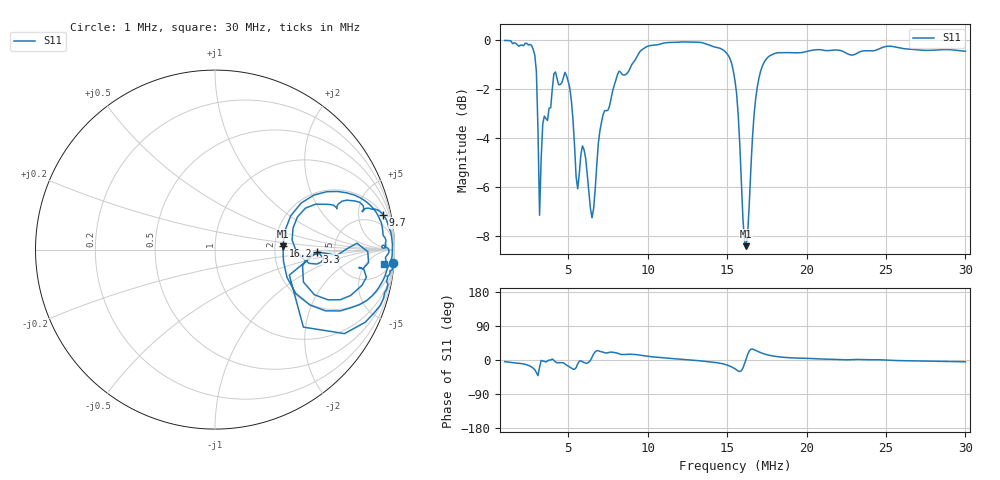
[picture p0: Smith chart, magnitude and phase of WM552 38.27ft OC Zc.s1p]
!Created via Zplots "Save as S1P" button
!Original data file:  $remote$.s1p
!Transmission line transform:  None
# MHZ S MA R 50
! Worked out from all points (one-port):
!   291 points, 1 MHz to 30 MHz, reference 50 ohm
!   lowest |S11| = -8.4 dB at 16.2 MHz (marker M1), VSWR 2.22, Z = 111 + j4.8 ohm
!   |S11| at or under -10 dB: nowhere
!   S11 on the Smith chart (normalised r, x): 1 MHz: 2, -27; 3.3 MHz: 3.65, -0.14; 9.7 MHz: 2.10, +9.36; 16.2 MHz: 2.21, +0.10; 30 MHz: 11, -17
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1  0.9957 -4.2
2.6  0.9773 -15.9
3  0.8601 -33.0
3.1  0.6549 -41.3
3.2  0.4379 -18.9
3.3  0.57 -1.3
4.1  0.8512 -0.7
4.7  0.8368 -7.6
5.3  0.6886 -24.0
5.5  0.5248 -20.2
5.7  0.5322 -3.3
5.9  0.6065 -4.7
6.2  0.5305 -8.3
6.5  0.4327 7.1
6.9  0.6146 24.3
8.3  0.858 14.9
9.7  0.9559 11.6
11.9  0.9873 2.8
14.7  0.9544 -9.8
15.5  0.8233 -23.2
15.8  0.6121 -30.3
16.2  0.3786 2.8
16.7  0.7024 27.4
17.5  0.9148 14.0
19.2  0.9396 5.4
22.8  0.9301 0.9
26.4  0.9561 -2.0
30  0.9465 -4.7
